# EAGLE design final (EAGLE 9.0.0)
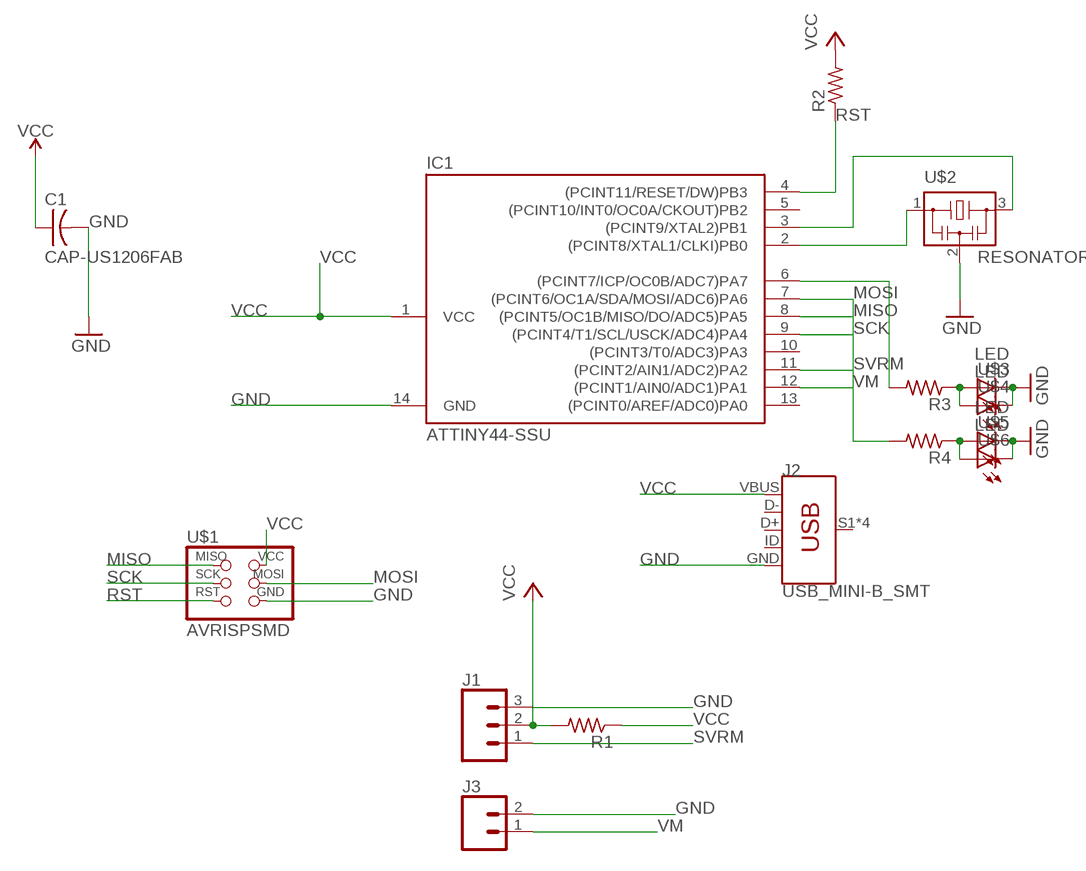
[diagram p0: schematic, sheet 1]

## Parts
C1  CAP-US1206FAB  [C1206FAB]
IC1  ATTINY44-SSU  [SOIC14]
J1  CONN_03LONGPADS  [1X03_LONGPADS]
J2  USB_MINI-B_SMT  [USB-MINIB]
J3  CONN_02PTH3  [1X02_LONGPADS]
R1  RES-US1206  [R1206]
R2  RES-US1206  [R1206]
R3  RES-US1206  [R1206]
R4  RES-US1206  [R1206]
U$1  AVRISPSMD  [2X03SMD]
U$2  RESONATOR  [EFOBM]
U$3  LED  [LED1206]
U$4  LED  [LED1206]
U$5  LED  [LED1206]
U$6  LED  [LED1206]

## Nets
GND: C1.2 IC1.14(GND) J1.3 J2.GND J3.2 U$1.6(GND) U$2.2 U$3.2(C) U$4.2(C) U$5.2(C) U$6.2(C)
MISO: IC1.8((PCINT5/OC1B/MISO/DO/ADC5)PA5) U$1.1(MISO)
MOSI: IC1.7((PCINT6/OC1A/SDA/MOSI/ADC6)PA6) R4.2 U$1.4(MOSI)
N$1: IC1.3((PCINT9/XTAL2)PB1) U$2.3
N$2: IC1.2((PCINT8/XTAL1/CLKI)PB0) U$2.1
N$4: R3.1 U$3.1(A) U$4.1(A)
N$5: R4.1 U$5.1(A) U$6.1(A)
N$6: IC1.6((PCINT7/ICP/OC0B/ADC7)PA7) R3.2
RST: IC1.4((PCINT11/RESET/DW)PB3) R2.1 U$1.5(RST)
SCK: IC1.9((PCINT4/T1/SCL/USCK/ADC4)PA4) U$1.3(SCK)
SVRM: IC1.11((PCINT2/AIN1/ADC2)PA2) J1.1
VCC: C1.1 IC1.1(VCC) J1.2 J2.VBUS R1.1 R1.2 R2.2 U$1.2(VCC)
VM: IC1.12((PCINT1/AIN0/ADC1)PA1) J3.1
Unconnected: IC1.5((PCINT10/INT0/OC0A/CKOUT)PB2) IC1.10((PCINT3/T0/ADC3)PA3) IC1.13((PCINT0/AREF/ADC0)PA0) J2.D+ J2.D- J2.ID J2.S1(SHIELD) J2.S2(SHIELD) J2.S3(SHIELD) J2.S4(SHIELD)

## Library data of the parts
C1 = fab:CAP-US
IC1 = fab:ATTINY44
J1 = SparkFun-Connectors:CONN_03: Multi connection point. Often used as Generic Header-pin footprint for 0.1 inch spaced/style header connections On any of the 0.1 inch spaced packages, you can populate with these: Break Away Headers - Straight (PRT-00116) Break Away Male Headers - Right Angle (PRT-00553) Female Headers (PRT-00115)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
J2 = SparkFun-Connectors:USB_MINI-B: USB type Mini-B Connector Breaks out 5th pin, and includes shield pins if needed. SparkFun Products: SparkFun FTDI Basic Breakout SparkFun XBee Explorer USB SparkFun Redboard; PROD_ID: CONN-08193; SF_ID: PRT-00587
J3 = SparkFun-Connectors:CONN_02: Multi connection point. Often used as Generic Header-pin footprint for 0.1 inch spaced/style header connections
R1-R4 = fab:RES-US: Resistor (US Symbol)
U$1 = fab:AVRISP
U$2 = fab:RESONATOR
U$3-U$6 = fab:LED: LED

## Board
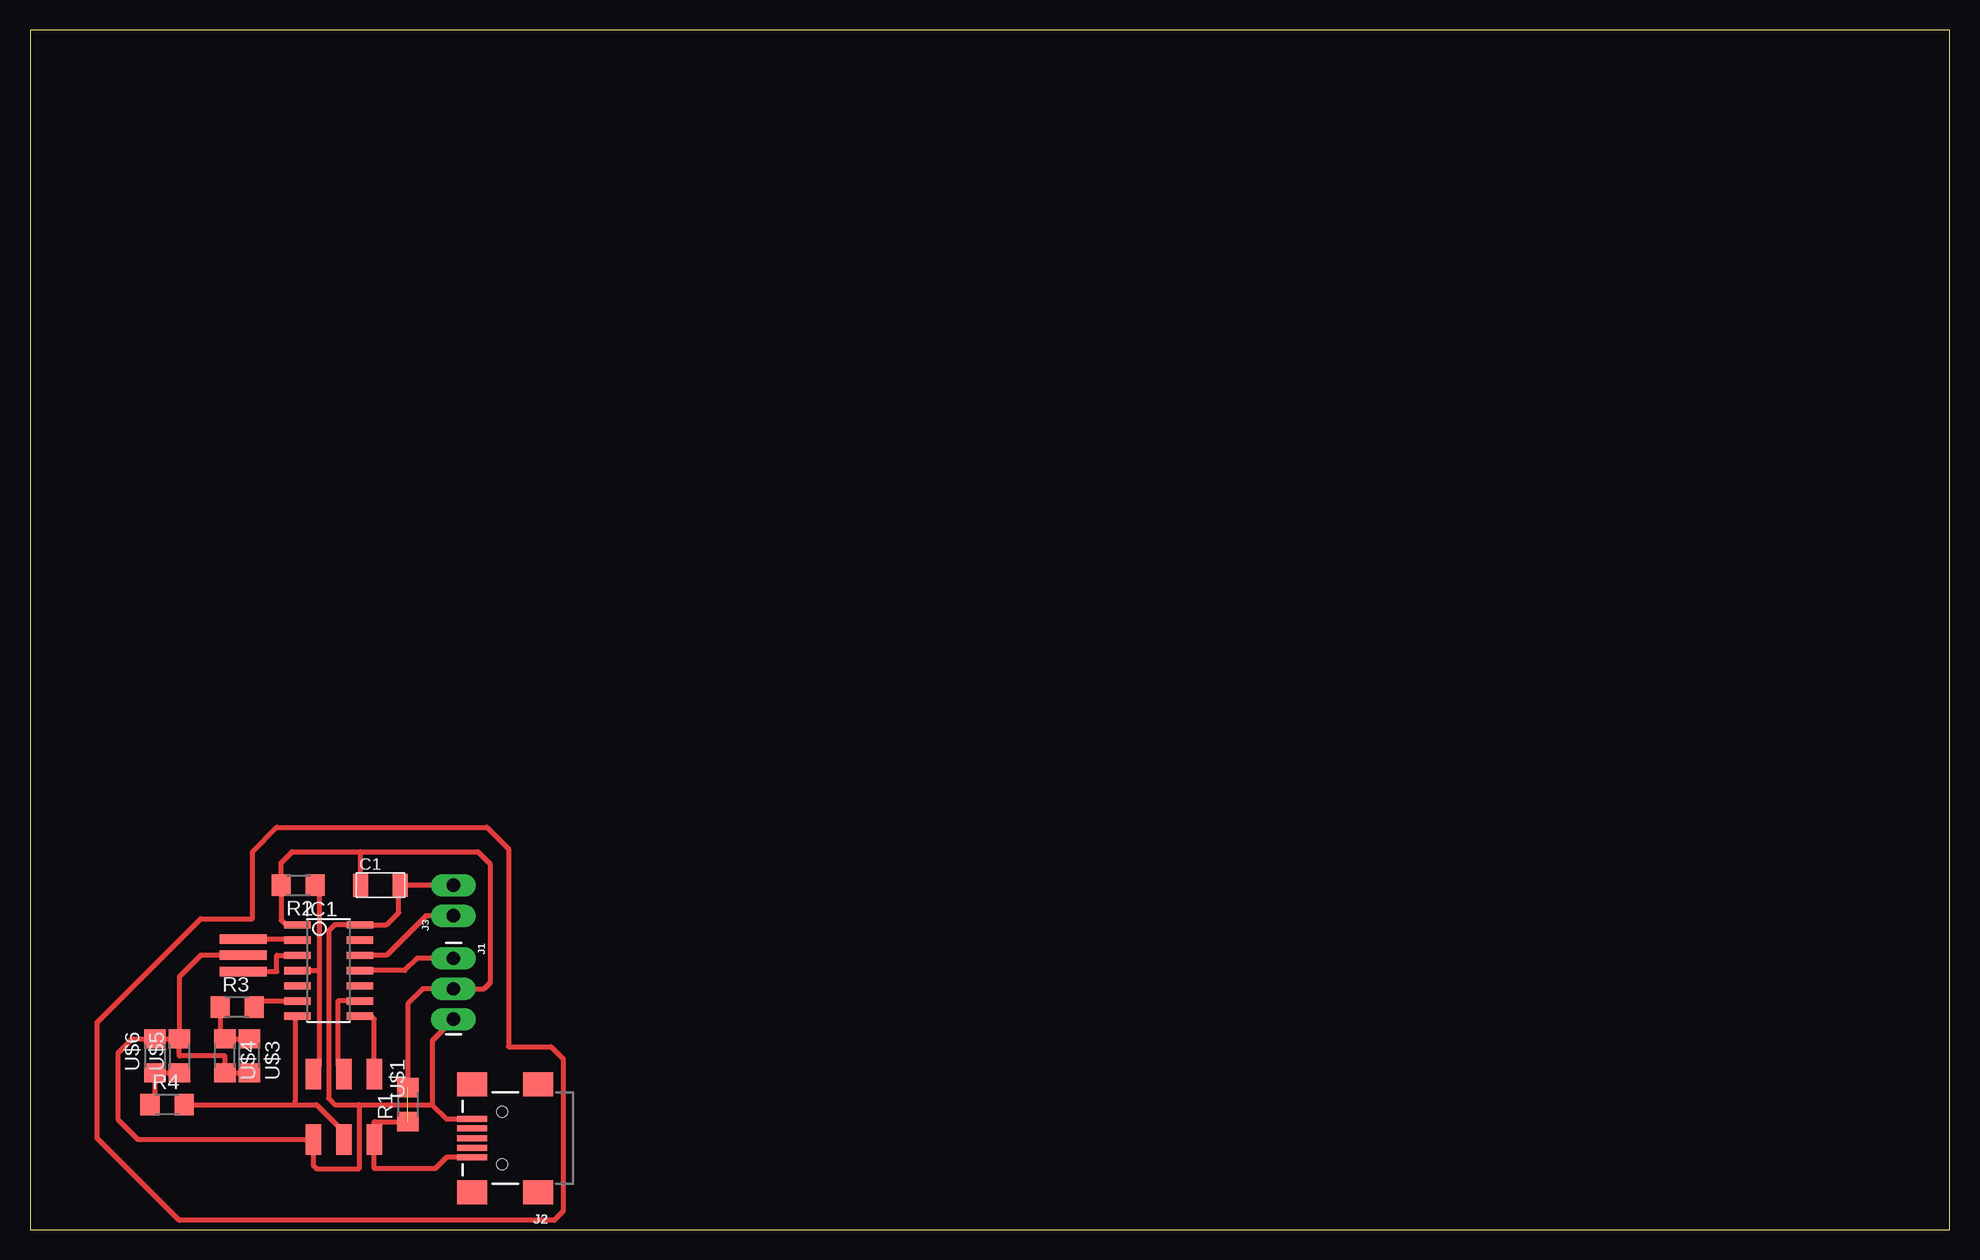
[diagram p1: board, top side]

Size 160 x 100 mm. Coordinates in mm from the lower left corner, seen from the top.
Outline: 0,0 160,0 160,100 0,100 0,0
Copper layers (1*16): Top 0.035mm / dielectric 1.5mm / Bottom 0.035mm
Design rules "default": minimum track width 6mil, minimum drill 0.35mm, track to track 6mil, track to pad 6mil, pad to pad 6mil, via to via 6mil, smd to smd 6mil, copper to edge 40mil, drill to drill 6mil, minimum pad ring 10mil, minimum via ring 8mil, stop-mask expansion 4mil, vias tented up to drill 0mil, thermal gap 10mil
bKeepout: 16 lines

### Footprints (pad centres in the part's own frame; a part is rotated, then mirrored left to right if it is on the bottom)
C1206FAB = smd 1.27 x 1.905: 1 -1.651,0; 2 1.651,0
SOIC14 = smd 0.61 x 2.21: 1 -3.81,-2.603; 2 -2.54,-2.603; 3 -1.27,-2.603; 4 0,-2.603; 5 1.27,-2.603; 6 2.54,-2.603; 7 3.81,-2.603; 8 3.81,2.603; 9 2.54,2.603; 10 1.27,2.603; 11 0,2.603; 12 -1.27,2.603; 13 -2.54,2.603; 14 -3.81,2.603
1X03_LONGPADS = drill 1.118 pad 1.88 long: 1 0,0; 2 2.54,0; 3 5.08,0
USB-MINIB = smd 2.5 x 0.5: D+ 2.5,0; D- 2.5,0.8; GND 2.5,-1.6; ID 2.5,-0.8; VBUS 2.5,1.6 | smd 2.5 x 2: S1 -3,4.5; S2 2.5,4.5; S3 -3,-4.5; S4 2.5,-4.5 | hole 0.9: 0,2.2; 0,-2.2
1X02_LONGPADS = drill 1.118 pad 1.88 long: 1 0,0; 2 2.54,0
R1206 = smd 1.6 x 1.803: 1 -1.422,0; 2 1.422,0
2X03SMD = smd 2.54 x 1.27: 1 -2.54,2.54; 2 2.92,2.54; 3 -2.54,0; 4 2.92,0; 5 -2.54,-2.54; 6 2.92,-2.54
EFOBM = smd 0.8 x 3.9: 1 -1.35,0; 2 0,0; 3 1.35,0
LED1206 = smd 1.6 x 1.803: 1 -1.422,0; 2 1.422,0

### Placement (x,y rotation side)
C1  29.21,28.7 0 top
IC1  24.89,21.59 270 top
J1  35.31,22.61 270 top
J2  39.37,7.62 180 top
J3  35.31,26.16 90 top
R1  31.5,10.41 90 top
R2  22.35,28.7 180 top
R3  17.27,18.54 0 top
R4  11.43,10.41 0 top
U$1  26.16,10.41 270 top
U$2  17.78,22.86 270 top
U$3  18.29,14.48 270 top
U$4  16.26,14.48 270 top
U$5  12.45,14.48 90 top
U$6  10.41,14.48 90 top

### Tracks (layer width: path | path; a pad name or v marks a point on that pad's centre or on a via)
GND
  Top 0.406: 27.43,10.41 27.43,5.08 23.88,5.08 23.62,5.33 U$1.6 9.02,7.49 7.37,9.14 7.37,14.73 8.53,15.9 U$6.2 U$5.2 | 27.43,10.41 33.53,10.41 | J3.2 C1.2 30.73,28.57 30.73,26.42 29.72,25.4 IC1.14 25.4,25.4 24.89,24.89 24.89,10.92 25.4,10.41 27.43,10.41 | 33.53,10.41 34.72,9.22 J2.GND | J1.3 33.53,15.75 33.53,10.41 | U$5.2 12.45,14.48 16.26,14.48 U$4.2 U$3.2 | U$2.2 14.22,22.86 12.45,21.08 U$5.2
MISO
  Top 0.406: U$1.1 28.7,17.53 28.45,17.78 IC1.8
MOSI
  Top 0.406: 25.91,7.75 U$1.4 26.16,8.13 23.88,10.41 22.1,10.41 | IC1.7 22.1,17.59 22.1,10.67 22.1,10.41 | 12.85,10.79 R4.2 22.1,10.41
N$1
  Top 0.406: U$2.3 20.57,21.51 20.57,22.86 IC1.3
N$2
  Top 0.406: U$2.1 22.21,24.21 IC1.2
N$3
  Top 0.406: 18.54,25.91 18.54,31.5 20.57,33.53 38.1,33.53 39.88,31.75 39.88,15.24 43.43,15.24 44.45,14.22 44.45,1.52 43.69,0.76 12.45,0.76 5.59,7.62 5.59,17.27 14.22,25.91 18.54,25.91
N$4
  Top 0.406: R3.1 15.85,15.9 U$4.1 U$3.1
N$5
  Top 0.406: U$5.1 U$6.1 10.41,10.41 R4.1
N$6
  Top 0.406: R3.2 18.69,19.05 IC1.6
RST
  Top 0.406: U$1.5 24.13,13.72 24.13,21.59 | 24.13,21.59 24.13,28.35 R2.1 | IC1.4 24.13,21.59
SCK
  Top 0.406: 26.06,13.01 U$1.3 | 25.91,13.16 26.06,13.01 | IC1.9 25.65,19.05 25.65,13.72 26.16,13.72 26.16,13.01 26.06,13.01
SVRM
  Top 0.406: J1.1 32.26,22.61 31.24,21.59 IC1.11
VCC  (1 unrouted)
  Top 0.406: 27.69,28.57 C1.1 27.56,31.5 | IC1.1 21.34,25.4 20.93,25.81 R2.2 20.93,30.58 21.84,31.5 27.56,31.5 | 27.56,31.5 37.34,31.5 38.35,30.48 38.35,20.57 37.85,20.07 J1.2 32.77,20.07 31.5,18.8 R1.2 | J2.VBUS 34.72,6.02 33.78,5.08 28.7,5.08 U$1.2 28.7,8.99 R1.1
VM
  Top 0.406: IC1.12 29.72,22.86 33.02,26.16 J3.1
